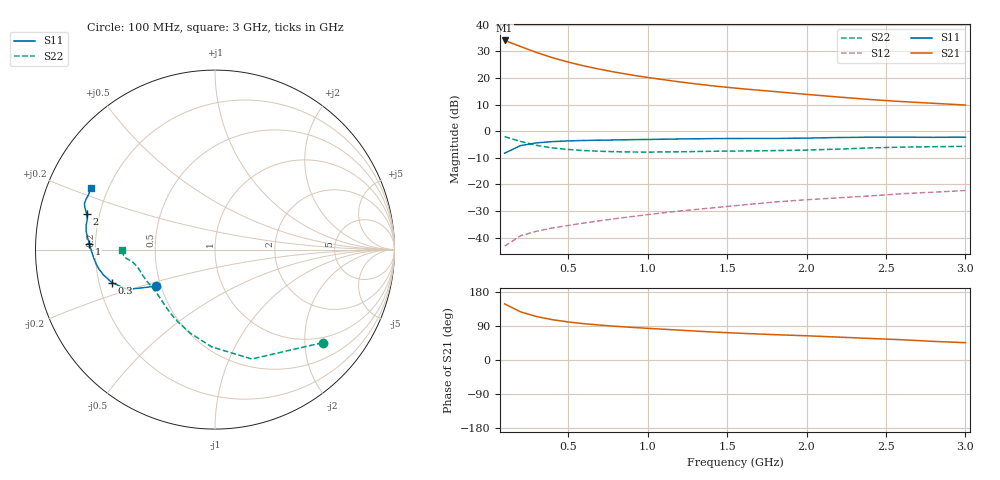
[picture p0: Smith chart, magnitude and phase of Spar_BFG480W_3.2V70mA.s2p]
! Filename: 3_270BFG480.001
! Title: BFG480W
! Bias: Vce=3.2V; Ic=70mA
! Company: NXP Semiconductors NL
! User: Quality&Reliability T&D
! Measure time: 10 Nov 1999 / 11:57:22
#  MHz  S  MA  R 50
! Freq  S11  S21  S12  S22  :
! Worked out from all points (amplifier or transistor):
!   20 points, 100 MHz to 3 GHz, reference 50 ohm
!   highest |S21| = 34.2 dB at 100 MHz (marker M1)
!   |S21| within 3 dB of that: start of sweep to 232.9 MHz
!   unconditionally stable (mu >= 1): 828 MHz to end of sweep
!   at 400 MHz: K = 0.74, MSG = 32.1 dB, |S12| = -36.4 dB
!   at 1.2 GHz: K = 1.07, MAG = 22.7 dB, |S12| = -30.0 dB
!   at 3 GHz: K = 1.06, MAG = 14.6 dB, |S12| = -22.3 dB
!   S11 on the Smith chart (normalised r, x): 100 MHz: 0.47, -0.23; 300 MHz: 0.25, -0.15; 1 GHz: 0.18, +0.02; 2 GHz: 0.15, +0.13; 3 GHz: 0.14, +0.23
100  0.3856 -148.1  51.02 148.0  0.006874 69.0  0.7924 -40.9
200  0.536 -155.5  39.34 127.2  0.01077 59.1  0.643 -71.4
300  0.6033 -162.3  30.35 114.7  0.01312 56.7  0.5425 -91.9
400  0.6374 -167.2  24.23 106.4  0.01507 57.4  0.486 -106.3
500  0.6573 -170.9  20.01 100.4  0.01684 59.3  0.4536 -116.8
600  0.6697 -173.8  16.92 95.8  0.01874 61.0  0.4334 -124.7
700  0.6782 -176.4  14.64 92.1  0.02068 63.2  0.42 -130.8
800  0.6854 -178.6  12.85 88.9  0.02269 65.0  0.4113 -135.9
900  0.6935 179.3  11.42 86.2  0.02475 67.0  0.4065 -140.4
1000  0.7003 177.4  10.27 83.6  0.02701 68.3  0.4052 -144.3
1200  0.715 174.2  8.484 78.8  0.03147 70.2  0.4105 -150.7
1400  0.7256 171.8  7.185 74.1  0.03591 71.6  0.4195 -155.4
1600  0.7308 169.4  6.269 70.2  0.04106 72.7  0.4252 -159.1
1800  0.7313 166.7  5.575 66.9  0.0466 73.5  0.4317 -162.9
2000  0.7419 164.4  4.936 63.9  0.05136 74.3  0.4424 -167.3
2200  0.7615 162.2  4.404 60.4  0.05574 74.4  0.4612 -171.0
2400  0.7719 160.5  3.949 56.8  0.06063 74.0  0.4849 -173.4
2600  0.7716 158.7  3.612 53.5  0.06664 73.5  0.5029 -174.9
2800  0.768 156.5  3.349 49.1  0.07133 72.2  0.5113 -176.8
3000  0.7726 153.8  3.11 45.7  0.07665 71.5  0.5186 -179.7
